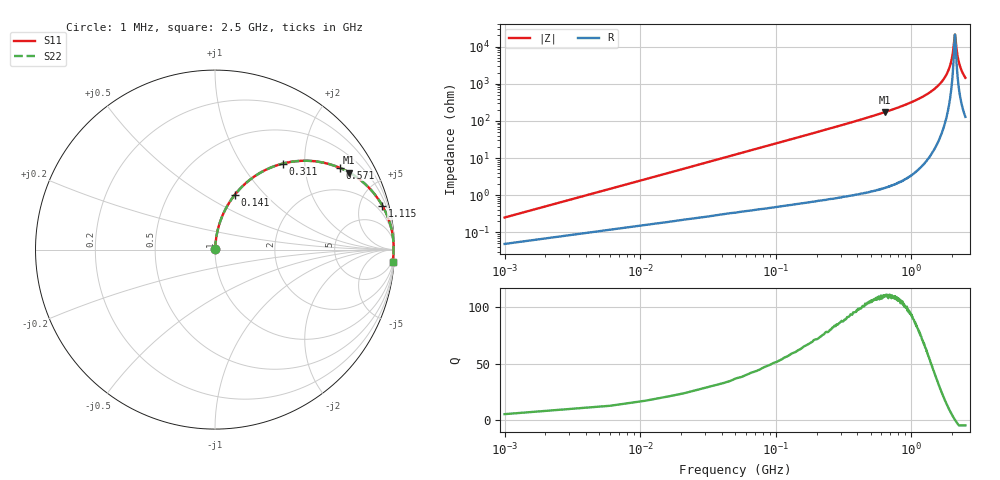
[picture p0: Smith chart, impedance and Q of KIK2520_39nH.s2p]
!version-2
!date-01.2022
!Series
# MHz S RI R 50
!Freq ReS11 ImS11 ReS21 ImS21 ReS12 ImS12 ReS22 ImS22
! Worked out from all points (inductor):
!   501 points, 1 MHz to 2.5 GHz, reference 50 ohm
!   read as one part in series: L = 39 nH near 11 MHz
!   highest Q = 110 at 641 MHz (marker M1), where L = 43 nH
!   self-resonance near 2.09 GHz
!   S11 on the Smith chart (normalised r, x): 1 MHz: 1.00, +0.00; 141 MHz: 1.01, +0.69; 311 MHz: 1.02, +1.56; 571 MHz: 1.03, +3.02; 1.115 GHz: 1.09, +7.64; 2.5 GHz: 4, -29
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1  0.000483 0.00245  0.9995 -0.00245  0.9995 -0.00245  0.000483 0.00245
16  0.00343 0.039  0.9966 -0.039  0.9966 -0.039  0.00343 0.039
36  0.0105 0.0871  0.9895 -0.0871  0.9895 -0.0871  0.0105 0.0871
76  0.0374 0.1788  0.9626 -0.1788  0.9626 -0.1788  0.0374 0.1788
141  0.1115 0.3066  0.8885 -0.3066  0.8885 -0.3066  0.1115 0.3066
311  0.3792 0.4795  0.6208 -0.4795  0.6208 -0.4795  0.3792 0.4795
421  0.5358 0.4937  0.4642 -0.4937  0.4642 -0.4937  0.5358 0.4937
571  0.6939 0.4563  0.3061 -0.4563  0.3061 -0.4563  0.6939 0.4563
641  0.7483 0.4295  0.2517 -0.4295  0.2517 -0.4295  0.7483 0.4295
836  0.8535 0.3489  0.1465 -0.3489  0.1465 -0.3489  0.8535 0.3489
1115  0.9332 0.2436  0.0668 -0.2436  0.0668 -0.2436  0.9332 0.2436
1255  0.9557 0.1983  0.0443 -0.1983  0.0443 -0.1983  0.9557 0.1983
1670  0.9886 0.0875  0.0114 -0.0875  0.0114 -0.0875  0.9886 0.0875
1830  0.9933 0.0521  0.0067 -0.0521  0.0067 -0.0521  0.9933 0.0521
1945  0.9949 0.0285  0.00508 -0.0285  0.00508 -0.0285  0.9949 0.0285
2020  0.9953 0.0139  0.00466 -0.0139  0.00466 -0.0139  0.9953 0.0139
2085  0.9953 0.00171  0.00467 -0.00171  0.00467 -0.00171  0.9953 0.00171
2105  0.9953 -0.00197  0.00473 0.00197  0.00473 0.00197  0.9953 -0.00197
2170  0.9949 -0.0137  0.00512 0.0137  0.00512 0.0137  0.9949 -0.0137
2245  0.9941 -0.0268  0.0059 0.0268  0.0059 0.0268  0.9941 -0.0268
2355  0.9924 -0.0452  0.00763 0.0452  0.00763 0.0452  0.9924 -0.0452
2500  0.9892 -0.0679  0.0108 0.0679  0.0108 0.0679  0.9892 -0.0679
